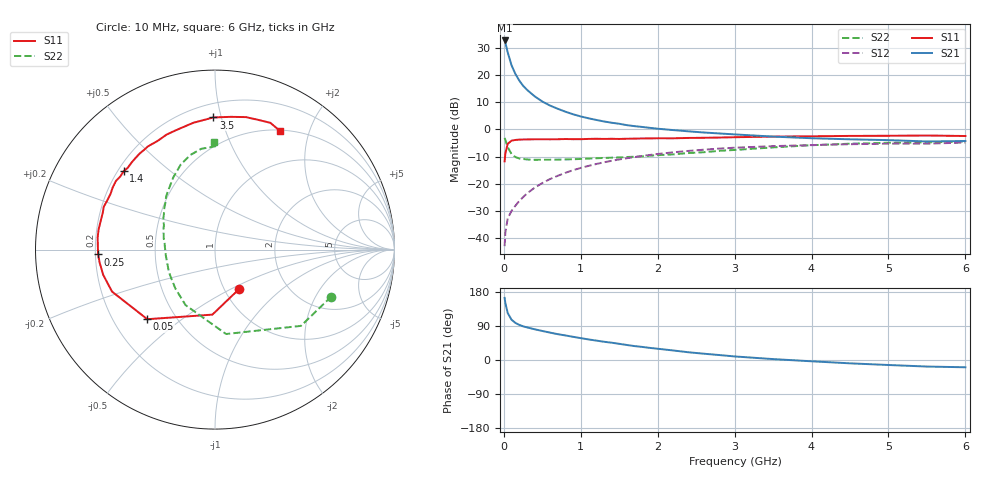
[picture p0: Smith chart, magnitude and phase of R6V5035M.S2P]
! SIEMENS Small Signal Semiconductors
! BFR193
! Si NPN RF Bipolar Junction Transistor in SOT23
! VCE = 0.5 V  IC = 35 mA
! Common Emitter S-Parameters:  May  1996
# GHz  S  MA  R  50
!  f  S11  S21  S12  S22
! GHz  MAG  ANG  MAG  ANG  MAG  ANG  MAG  ANG
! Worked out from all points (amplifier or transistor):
!   36 points, 10 MHz to 6 GHz, reference 50 ohm
!   highest |S21| = 32.7 dB at 10 MHz (marker M1)
!   |S21| within 3 dB of that: start of sweep to 38.5 MHz
!   unconditionally stable (mu >= 1): 229.1 MHz to end of sweep
!   at 250 MHz: K = 1.02, MAG = 19.6 dB, |S12| = -24.9 dB
!   at 1.4 GHz: K = 1.08, MAG = 5.3 dB, |S12| = -11.6 dB
!   at 6 GHz: K = 1.02, MAG = -0.6 dB, |S12| = -4.9 dB
!   S11 on the Smith chart (normalised r, x): 10 MHz: 1.16, -0.55; 50 MHz: 0.35, -0.38; 250 MHz: 0.21, -0.02; 1.4 GHz: 0.22, +0.35; 3.5 GHz: 0.29, +0.94; 6 GHz: 0.51, +1.56
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0.01  0.2583 -59.3  43.2 163.8  0.0071 73.6  0.6988 -22.0
0.02  0.3626 -92.3  39.29 149.9  0.0127 68.9  0.6402 -41.6
0.05  0.541 -134.2  26.17 124.1  0.0229 54.8  0.4744 -82.5
0.1  0.6195 -157.8  15.1 106.3  0.0316 54.9  0.3502 -117.9
0.15  0.6388 -167.3  10.47 97.9  0.0394 57.9  0.3095 -135.5
0.2  0.6467 -173.5  7.928 92.7  0.048 61.9  0.2916 -146.6
0.25  0.6515 -177.6  6.349 88.9  0.0567 63.8  0.2851 -154.6
0.3  0.6525 179.4  5.352 86.1  0.066 65.8  0.2795 -159.6
0.4  0.6573 174.0  4.059 81.1  0.0844 67.0  0.2756 -167.0
0.5  0.6581 170.1  3.251 76.6  0.1029 67.2  0.2759 -172.9
0.6  0.6565 165.5  2.743 72.3  0.1219 66.6  0.2768 -177.0
0.7  0.6582 161.8  2.393 68.2  0.1398 65.7  0.2776 179.8
0.9  0.6596 155.0  1.895 61.2  0.1774 63.0  0.2818 173.6
1.1  0.667 148.7  1.599 54.3  0.2127 59.7  0.2904 168.8
1.4  0.6707 139.3  1.325 45.7  0.2639 54.4  0.3015 161.9
1.7  0.6757 130.9  1.145 36.7  0.309 49.0  0.3137 155.2
2.2  0.6847 117.9  0.97 25.2  0.3782 39.7  0.3466 145.2
2.8  0.707 103.6  0.841 13.1  0.4433 28.9  0.4029 132.5
3.5  0.7364 90.7  0.736 2.4  0.4915 17.1  0.4658 119.8
4.5  0.7579 76.9  0.656 -8.8  0.5331 3.7  0.5449 104.5
5.5  0.7708 66.4  0.599 -17.3  0.5454 -8.3  0.5756 89.8
6  0.7542 61.4  0.61 -19.2  0.5717 -12.1  0.5992 90.5
